(* Logix 5000 Routine export ControlNetRouter; software revision 19.01 *)

TYPE AparianCNROutput :
STRUCT
   GeneralCtrl : DINT;
   MappedData : SINT[400];
END_STRUCT
END_TYPE

TYPE AparianCNREInput :
STRUCT
   GeneralStatus : SINT;
   CNetNodeNumber : SINT;
   CNetLedState : SINT;
   CNetMode : SINT;
   Temperature : REAL;
   MappedData : SINT[492];
END_STRUCT
END_TYPE

TYPE AparianCNRInput :
STRUCT
   GeneralStatus : SINT;
   CNetNodeNumber : SINT;
   CNetLedState : SINT;
   CNetMode : SINT;
   Temperature : REAL;
   MappedData : SINT[400];
END_STRUCT
END_TYPE

TYPE AparianCNREOutput :
STRUCT
   GeneralCtrl : DINT;
   MappedData : SINT[492];
END_STRUCT
END_TYPE

VAR_GLOBAL   (* controller tags *)
   CNR01Output : AparianCNROutput;
   eCNR01Input1 : AparianCNREInput;
   CNR01Input : AparianCNRInput;
   eCNR01Output1 : AparianCNREOutput;
END_VAR

PROGRAM MainProgram

ROUTINE ControlNetRouter   (* ladder *)
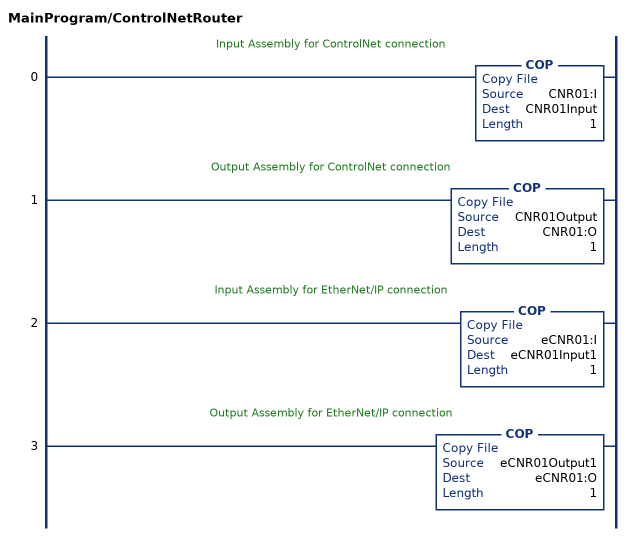
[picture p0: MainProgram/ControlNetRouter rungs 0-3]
   // Input Assembly for ControlNet connection
   0: COP(CNR01:I,CNR01Input,1);
   // Output Assembly for ControlNet connection
   1: COP(CNR01Output,CNR01:O,1);
   // Input Assembly for EtherNet/IP connection
   2: COP(eCNR01:I,eCNR01Input1,1);
   // Output Assembly for EtherNet/IP connection
   3: COP(eCNR01Output1,eCNR01:O,1);
END_ROUTINE
END_PROGRAM
